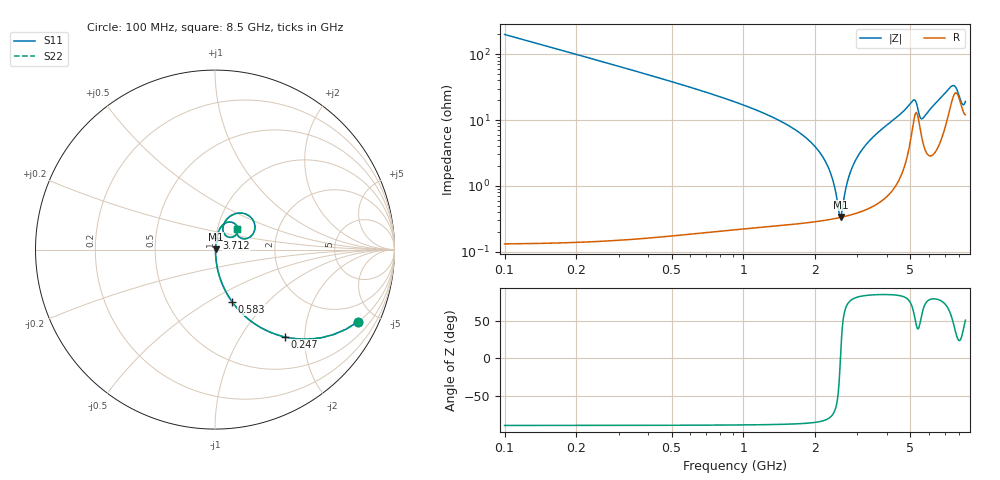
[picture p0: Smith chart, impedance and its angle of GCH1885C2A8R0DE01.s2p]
!Murata Part Number: GCH1885C2A8R0DE01
!These Parameters are Measured in Series Mode Connection
!Data Generated on Jun 19, 2026
!  o--ll--o
!Port1  Port2
!  o------o
!Operation Temp=25[degC], DC Bias Voltage=0[V]
!Freq. Start=100[MHz] Stop=9[GHz] 401[Steps]
# Hz S RI R 50
!Freq.(Hz) S11(Real) S11(Imag) S21(Real) S21(Imag) S12(Real) S12(Imag) S22(Real) S22(Imag)
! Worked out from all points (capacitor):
!   401 points, 100 MHz to 8.5 GHz, reference 50 ohm
!   read as one part in series: C = 8 pF near 142 MHz
!   lowest |Z| = 338 mohm at 2.557 GHz (marker M1)
!   series resonance near 2.548 GHz, so ESL is about 490 pH
!   S11 on the Smith chart (normalised r, x): 100 MHz: 1.00, -3.97; 247 MHz: 1.00, -1.60; 583 MHz: 1.00, -0.65; 3.712 GHz: 1.01, +0.14; 8.5 GHz: 1.24, +0.30
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1e8  0.7976 -0.4014  0.2024 0.4014  0.2024 0.4014  0.7976 -0.4014
2.47e8  0.3891 -0.4867  0.6109 0.4867  0.6109 0.4867  0.3891 -0.4867
3.94e8  0.1962 -0.3955  0.8038 0.3955  0.8038 0.3955  0.1962 -0.3955
5.83e8  0.0961 -0.2919  0.9039 0.2919  0.9039 0.2919  0.0961 -0.2919
1.507e9  0.00996 -0.0857  0.99 0.0857  0.99 0.0857  0.00996 -0.0857
1.906e9  0.00497 -0.0465  0.995 0.0465  0.995 0.0465  0.00497 -0.0465
2.179e9  0.00362 -0.025  0.9964 0.025  0.9964 0.025  0.00362 -0.025
2.347e9  0.0033 -0.0132  0.9967 0.0132  0.9967 0.0132  0.0033 -0.0132
2.515e9  0.00328 -0.00209  0.9967 0.00209  0.9967 0.00209  0.00328 -0.00209
2.557e9  0.00332 0.00058  0.9967 -0.00058  0.9967 -0.00058  0.00332 0.00058
2.725e9  0.00363 0.0109  0.9964 -0.0109  0.9964 -0.0109  0.00363 0.0109
2.914e9  0.00424 0.0221  0.9958 -0.0221  0.9958 -0.0221  0.00424 0.0221
3.229e9  0.00588 0.0399  0.9941 -0.0399  0.9941 -0.0399  0.00588 0.0399
3.712e9  0.01 0.0665  0.99 -0.0665  0.99 -0.0665  0.01 0.0665
4.3e9  0.0198 0.101  0.9802 -0.101  0.9802 -0.101  0.0198 0.101
5.161e9  0.1105 0.1441  0.8895 -0.1441  0.8895 -0.1441  0.1105 0.1441
5.497e9  0.0737 0.0703  0.9263 -0.0703  0.9263 -0.0703  0.0737 0.0703
5.707e9  0.0474 0.0957  0.9526 -0.0957  0.9526 -0.0957  0.0474 0.0957
7.114e9  0.1369 0.2037  0.8631 -0.2037  0.8631 -0.2037  0.1369 0.2037
7.702e9  0.2226 0.1209  0.7774 -0.1209  0.7774 -0.1209  0.2226 0.1209
8.227e9  0.1377 0.0679  0.8623 -0.0679  0.8623 -0.0679  0.1377 0.0679
8.5e9  0.1228 0.1162  0.8772 -0.1162  0.8772 -0.1162  0.1228 0.1162
